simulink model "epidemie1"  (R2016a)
settings: Solver=FixedStepDiscrete  StartTime=0.0  StopTime=300  FixedStep=1  RelTol=1e-3
InitFcn:
  | init_epidemie
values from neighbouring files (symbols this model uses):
  alpha = 2e-6    (= 2e-06)    [init_epidemie.m]
  b0 = 5e3    (= 5000)    [init_epidemie.m]
  beta = 1    [init_epidemie.m]
  delta = 0.1    [init_epidemie.m]
  gamma = 0.9    [init_epidemie.m]

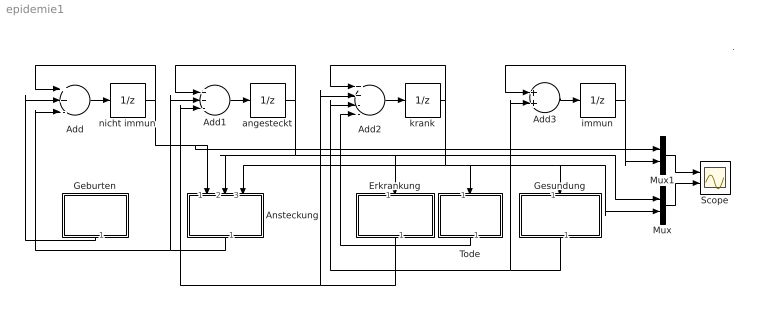
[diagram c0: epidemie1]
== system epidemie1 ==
  note: .
  Add : Sum  Inputs=++-
  Add1 : Sum  Inputs=++-
  Add2 : Sum  Inputs=++--
  Add3 : Sum
  Ansteckung : Subsystem
  Erkrankung : Subsystem
  Geburten : Subsystem
  Gesundung : Subsystem
  Mux : Mux  Inputs=2
  Mux1 : Mux  Inputs=2
  Scope : Scope  NumInputPorts=2
  Tode : Subsystem
  angesteckt : UnitDelay  InitialCondition=1  SampleTime=-1
  immun : UnitDelay  SampleTime=-1
  krank : UnitDelay  SampleTime=-1
  nicht immun : UnitDelay  InitialCondition=1e6  SampleTime=-1
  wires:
  Add/1 -> nicht immun/1
  nicht immun/1 -> Add/1, Ansteckung/1(N), Mux1/1
  immun/1 -> Add3/1, Mux1/2
  Geburten/1(b) -> Add/2
  angesteckt/1 -> Add1/1, Ansteckung/2(A), Erkrankung/1(A), Mux/1
  krank/1 -> Ansteckung/3(K), Tode/1(K), Gesundung/1(K), Mux/2, Add2/1
  Ansteckung/1(a) -> Add/3, Add1/2
  Add1/1 -> angesteckt/1
  Erkrankung/1(k) -> Add1/3, Add2/2
  Add2/1 -> krank/1
  Gesundung/1(g) -> Add2/3, Add3/2
  Add3/1 -> immun/1
  Tode/1(t) -> Add2/4
  Mux1/1 -> Scope/1
  Mux/1 -> Scope/2

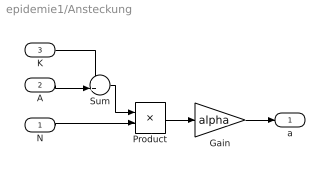
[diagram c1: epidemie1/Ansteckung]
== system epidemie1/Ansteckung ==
  N : Inport
  A : Inport  Port=2
  K : Inport  Port=3
  Gain : Gain  Gain=alpha
  Product : Product
  Sum : Sum  Inputs=++|
  a : Outport
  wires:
  Sum/1 -> Product/1
  Product/1 -> Gain/1
  K/1 -> Sum/1
  A/1 -> Sum/2
  Gain/1 -> a/1
  N/1 -> Product/2

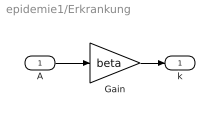
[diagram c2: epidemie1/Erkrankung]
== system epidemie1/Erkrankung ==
  A : Inport
  Gain : Gain  Gain=beta
  k : Outport
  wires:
  A/1 -> Gain/1
  Gain/1 -> k/1

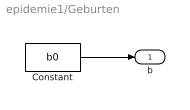
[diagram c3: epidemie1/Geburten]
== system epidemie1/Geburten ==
  Constant : Constant  Value=b0
  b : Outport
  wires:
  Constant/1 -> b/1

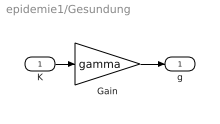
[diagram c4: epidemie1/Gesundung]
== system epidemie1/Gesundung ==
  K : Inport
  Gain : Gain  Gain=gamma
  g : Outport
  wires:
  Gain/1 -> g/1
  K/1 -> Gain/1

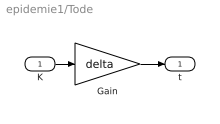
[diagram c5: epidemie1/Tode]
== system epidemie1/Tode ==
  K : Inport
  Gain : Gain  Gain=delta
  t : Outport
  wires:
  K/1 -> Gain/1
  Gain/1 -> t/1
